(* Logix 5000 AddOnInstructionDefinition export Banner_IOLM_Param_A2_v6; software revision 36.05 *)

TYPE Banner_IOL_Port_v6 :   // UDT that has all of the data items necessary to communicate with a specific Port on a IO-Link Master
STRUCT
   Port_Controlled : INT;   // Each bit represents a port on an IO-Link Master. Set to 1 to tell AOI to control that port.
   Port_Activate : INT;   // Each bit represents a port on an IO-Link Master. When ON that port will process any commands in queue.
   Port_Read : INT;   // Each bit represents a port on an IO-Link Master. Used to determine when device AOI has requested a Read command.
   Port_Write : INT;   // Each bit represents a port on an IO-Link Master. Used to determine when device AOI has requested a Write command.
   Port_RW_Complete : INT;   // Each bit represents a port on an IO-Link Master. Tells device AOI that Read or Write request has been completed.
   Port_Device_Read : INT;
   Data_Transfer : SINT[250];   // Array to transfer data from IO-Master to device AOIs.
END_STRUCT
END_TYPE

TYPE Banner_IOLM_EL_v6 :   // Error Log for Messages to IOLM.
STRUCT
   RW : SINT;   // 0 = Read, 1 = Write.
   Port : SINT;   // Port number that generated error.
   Index : INT;   // IO-Link Index for generated error.
END_STRUCT
END_TYPE

TYPE Banner_IOLM_v6 :   // UDT to control IO-Link Masters.
STRUCT
   Message_Source_Data : SINT[260];
   Message_Destination_Data : SINT[260];
   Error_Log : Banner_IOLM_EL_v6[10];
   Error_Write_Retry : BOOL;
   Num_Error_MSGS : DINT;
   IO_Link_Master_Busy : BOOL;   // 0 = While waiting for a command, 1 = Processing command
   AOI_Reset : BOOL;
   Port_Data : Banner_IOL_Port_v6;   // All of the necessary data to work with the various ports of the IO-Link Master.
   Halt_Operation : BOOL;   // When parameter is 1 the AOI is halted as next available time frame.
   AOI_Halted : BOOL;   // AOI is in standby mode until Halt Operation tag is set back to 0.
END_STRUCT
END_TYPE

ADD_ON_INSTRUCTION Banner_IOLM_Param_A2_v6   (* revision 6.0, vendor Banner Engineering *)
// AOI that controls an Allen Bradley IO-Link Master with Banner devices for parameter data operations. Created for use with the 5032-8IOLM units only.
VAR_IN_OUT
   Message_Read : MESSAGE; {required}   // Message used to gather data from a device plugged into an Allen Bradley IO-Link Master.
   Message_Write : MESSAGE; {required}   // Message used to send parameter updates to a device plugged into an Allen Bradley IO-Link Master.
   IOLM : Banner_IOLM_v6; {required}
   ISDU_Path : STRING[8]; {required}
END_VAR
VAR_INPUT
   Port0 : BOOL; {required}
   Port1 : BOOL; {required}
   Port2 : BOOL; {required}
   Port3 : BOOL; {required}
   Port4 : BOOL; {required}
   Port5 : BOOL; {required}
   Port6 : BOOL; {required}
   Port7 : BOOL; {required}
END_VAR
VAR_OUTPUT
   Done : BOOL; {access Read Only, visible}
   Busy : BOOL; {access Read Only, visible}
   Error : BOOL; {access Read Only, visible}
END_VAR
VAR
   Lock : DINT; {access None}
   Byte_Length : SINT; {access None}
   Current_Port : INT; {access None}   // Current port to communicate with via the IO-Link Master.
   Array_Index : DINT; {access None}
   Data_Index : DINT; {access None}
   Message_Timer : TIMER := (PRE := 100); {access None}
   Error_Index : DINT; {access None}
   Message_Timer2 : TIMER := (PRE := 5000); {access None}
   Temp_Index : INT; {access None}
   Timer8 : TIMER := (PRE := 3000); {access None}
END_VAR

ROUTINE Logic   (* ladder *)
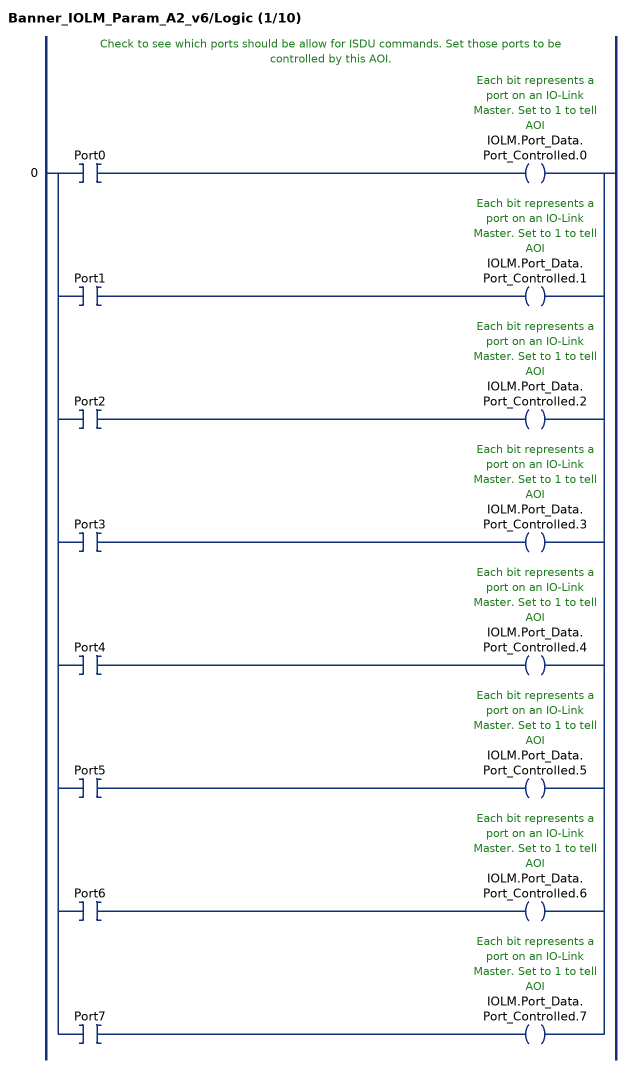
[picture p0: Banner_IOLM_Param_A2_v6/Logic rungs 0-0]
   // Check to see which ports should be allow for ISDU commands. Set those ports to be controlled by this AOI.
   0: [XIC(Port0) OTE(IOLM.Port_Data.Port_Controlled.0) ,XIC(Port1) OTE(IOLM.Port_Data.Port_Controlled.1) ,XIC(Port2) OTE(IOLM.Port_Data.Port_Controlled.2) ,XIC(Port3) OTE(IOLM.Port_Data.Port_Controlled.3) ,XIC(Port4) OTE(IOLM.Port_Data.Port_Controlled.4) ,XIC(Port5) OTE(IOLM.Port_Data.Port_Controlled.5) ,XIC(Port6) OTE(IOLM.Port_Data.Port_Controlled.6) ,XIC(Port7) OTE(IOLM.Port_Data.Port_Controlled.7) ];
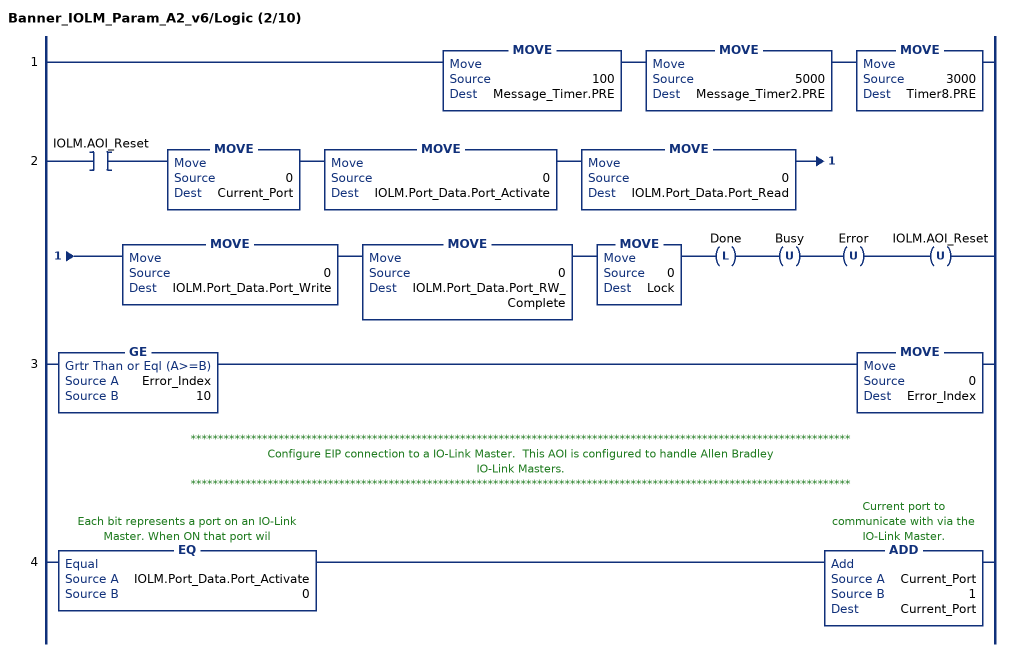
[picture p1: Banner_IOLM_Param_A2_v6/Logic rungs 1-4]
   1: MOVE(100,Message_Timer.PRE)MOVE(5000,Message_Timer2.PRE)MOVE(3000,Timer8.PRE);
   2: XIC(IOLM.AOI_Reset)MOVE(0,Current_Port)MOVE(0,IOLM.Port_Data.Port_Activate)MOVE(0,IOLM.Port_Data.Port_Read)MOVE(0,IOLM.Port_Data.Port_Write)MOVE(0,IOLM.Port_Data.Port_RW_Complete)MOVE(0,Lock)OTL(Done)OTU(Busy)OTU(Error)OTU(IOLM.AOI_Reset);
   3: GE(Error_Index,10)MOVE(0,Error_Index);
   // ************************************************************************************************************************
   // Configure EIP connection to a IO-Link Master.  This AOI is configured to handle Allen Bradley
   // IO-Link Masters.
   // ************************************************************************************************************************
   4: EQ(IOLM.Port_Data.Port_Activate,0)ADD(Current_Port,1,Current_Port);
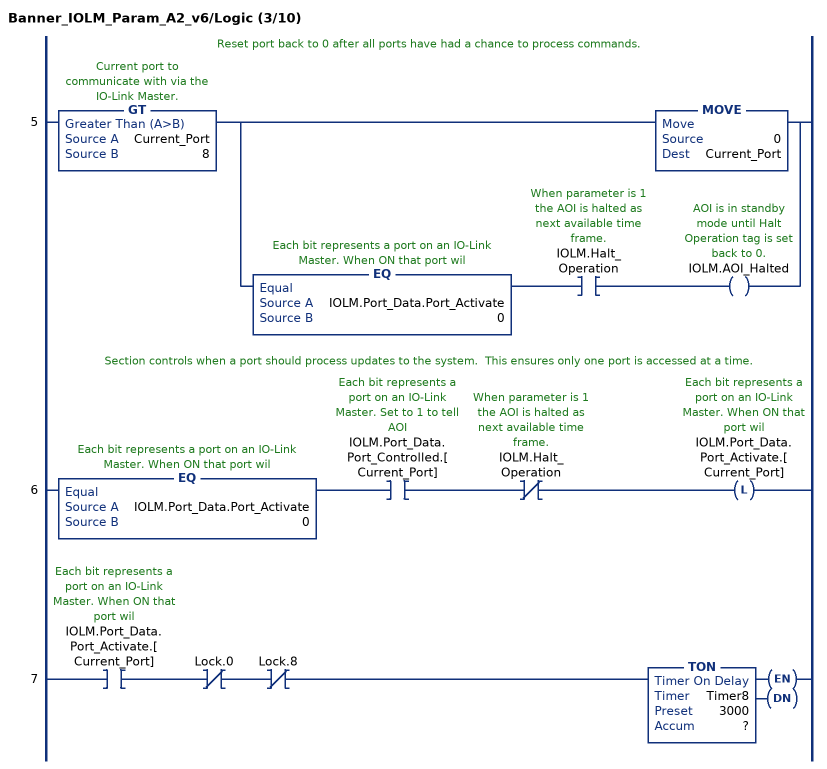
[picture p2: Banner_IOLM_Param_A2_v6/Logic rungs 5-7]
   // Reset port back to 0 after all ports have had a chance to process commands.
   5: GT(Current_Port,8)[MOVE(0,Current_Port) ,EQ(IOLM.Port_Data.Port_Activate,0) XIC(IOLM.Halt_Operation) OTE(IOLM.AOI_Halted) ];
   // Section controls when a port should process updates to the system.  This ensures only one port is accessed at a time.
   6: EQ(IOLM.Port_Data.Port_Activate,0)XIC(IOLM.Port_Data.Port_Controlled.[Current_Port])XIO(IOLM.Halt_Operation)OTL(IOLM.Port_Data.Port_Activate.[Current_Port]);
   7: XIC(IOLM.Port_Data.Port_Activate.[Current_Port])XIO(Lock.0)XIO(Lock.8)TON(Timer8,?,?);
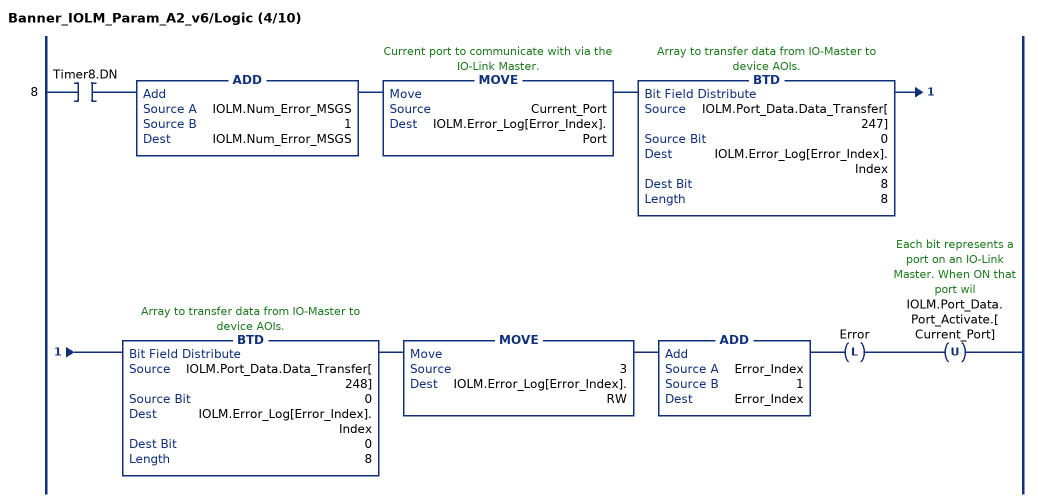
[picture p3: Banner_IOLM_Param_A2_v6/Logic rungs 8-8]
   8: XIC(Timer8.DN)ADD(IOLM.Num_Error_MSGS,1,IOLM.Num_Error_MSGS)MOVE(Current_Port,IOLM.Error_Log[Error_Index].Port)BTD(IOLM.Port_Data.Data_Transfer[247],0,IOLM.Error_Log[Error_Index].Index,8,8)BTD(IOLM.Port_Data.Data_Transfer[248],0,IOLM.Error_Log[Error_Index].Index,0,8)MOVE(3,IOLM.Error_Log[Error_Index].RW)ADD(Error_Index,1,Error_Index)OTL(Error)OTU(IOLM.Port_Data.Port_Activate.[Current_Port]);
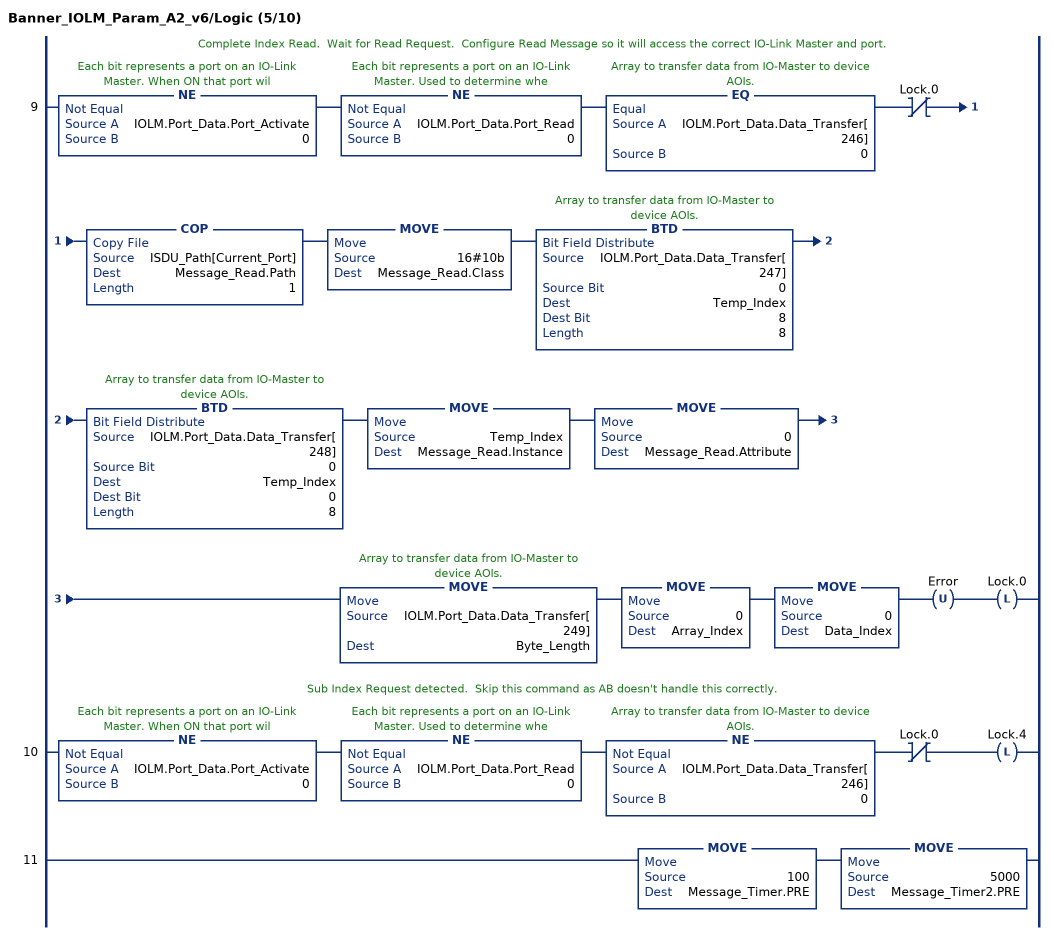
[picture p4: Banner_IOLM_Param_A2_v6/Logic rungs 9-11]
   // Complete Index Read.  Wait for Read Request.  Configure Read Message so it will access the correct IO-Link Master and port.
   9: NE(IOLM.Port_Data.Port_Activate,0)NE(IOLM.Port_Data.Port_Read,0)EQ(IOLM.Port_Data.Data_Transfer[246],0)XIO(Lock.0)COP(ISDU_Path[Current_Port],Message_Read.Path,1)MOVE(16#10b,Message_Read.Class)BTD(IOLM.Port_Data.Data_Transfer[247],0,Temp_Index,8,8)BTD(IOLM.Port_Data.Data_Transfer[248],0,Temp_Index,0,8)MOVE(Temp_Index,Message_Read.Instance)MOVE(0,Message_Read.Attribute)MOVE(IOLM.Port_Data.Data_Transfer[249],Byte_Length)MOVE(0,Array_Index)MOVE(0,Data_Index)OTU(Error)OTL(Lock.0);
   // Sub Index Request detected.  Skip this command as AB doesn't handle this correctly.
   10: NE(IOLM.Port_Data.Port_Activate,0)NE(IOLM.Port_Data.Port_Read,0)NE(IOLM.Port_Data.Data_Transfer[246],0)XIO(Lock.0)OTL(Lock.4);
   11: MOVE(100,Message_Timer.PRE)MOVE(5000,Message_Timer2.PRE);
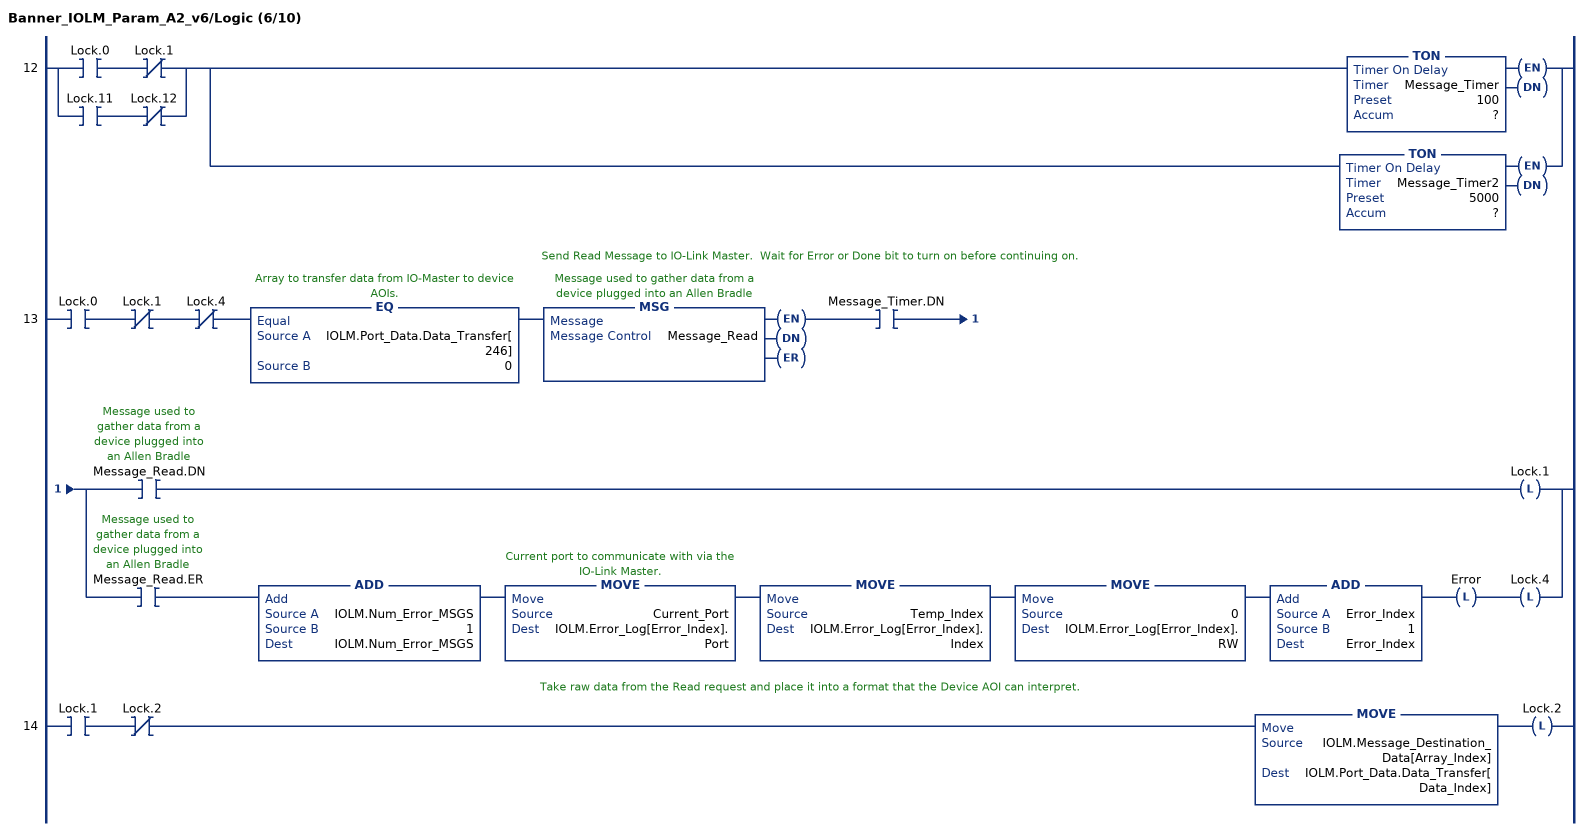
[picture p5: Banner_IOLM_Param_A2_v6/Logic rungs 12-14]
   12: [XIC(Lock.0) XIO(Lock.1) ,XIC(Lock.11) XIO(Lock.12) ][TON(Message_Timer,?,?) ,TON(Message_Timer2,?,?) ];
   // Send Read Message to IO-Link Master.  Wait for Error or Done bit to turn on before continuing on.
   13: XIC(Lock.0)XIO(Lock.1)XIO(Lock.4)EQ(IOLM.Port_Data.Data_Transfer[246],0)MSG(Message_Read)XIC(Message_Timer.DN)[XIC(Message_Read.DN) OTL(Lock.1) ,XIC(Message_Read.ER) ADD(IOLM.Num_Error_MSGS,1,IOLM.Num_Error_MSGS) MOVE(Current_Port,IOLM.Error_Log[Error_Index].Port) MOVE(Temp_Index,IOLM.Error_Log[Error_Index].Index) MOVE(0,IOLM.Error_Log[Error_Index].RW) ADD(Error_Index,1,Error_Index) OTL(Error) OTL(Lock.4) ];
   // Take raw data from the Read request and place it into a format that the Device AOI can interpret.
   14: XIC(Lock.1)XIO(Lock.2)MOVE(IOLM.Message_Destination_Data[Array_Index],IOLM.Port_Data.Data_Transfer[Data_Index])OTL(Lock.2);
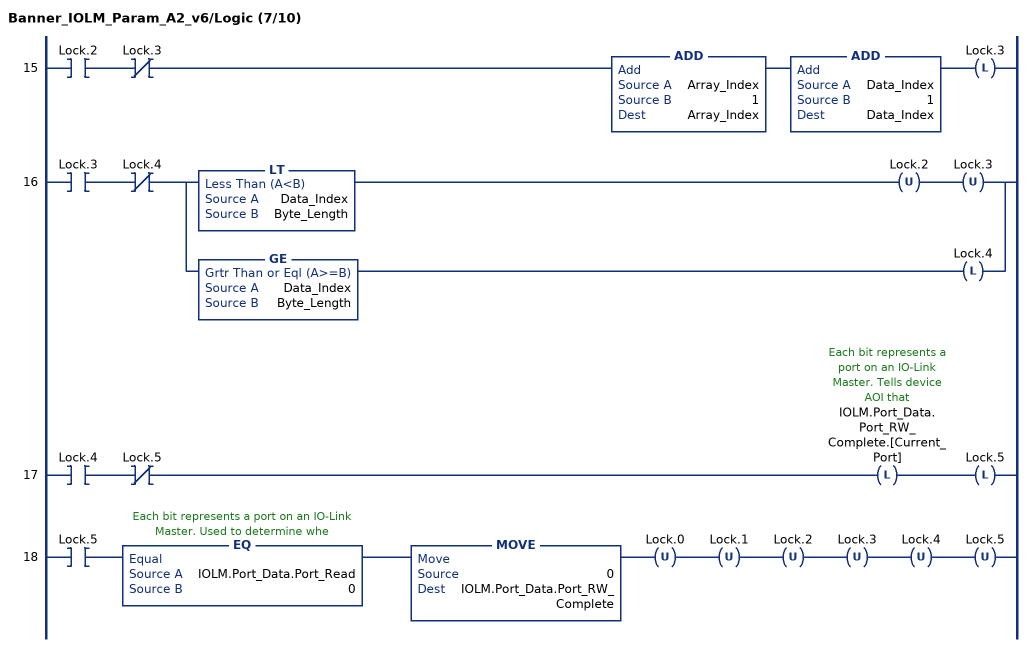
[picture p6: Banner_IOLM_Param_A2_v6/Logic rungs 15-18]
   15: XIC(Lock.2)XIO(Lock.3)ADD(Array_Index,1,Array_Index)ADD(Data_Index,1,Data_Index)OTL(Lock.3);
   16: XIC(Lock.3)XIO(Lock.4)[LT(Data_Index,Byte_Length) OTU(Lock.2) OTU(Lock.3) ,GE(Data_Index,Byte_Length) OTL(Lock.4) ];
   17: XIC(Lock.4)XIO(Lock.5)OTL(IOLM.Port_Data.Port_RW_Complete.[Current_Port])OTL(Lock.5);
   18: XIC(Lock.5)EQ(IOLM.Port_Data.Port_Read,0)MOVE(0,IOLM.Port_Data.Port_RW_Complete)OTU(Lock.0)OTU(Lock.1)OTU(Lock.2)OTU(Lock.3)OTU(Lock.4)OTU(Lock.5);
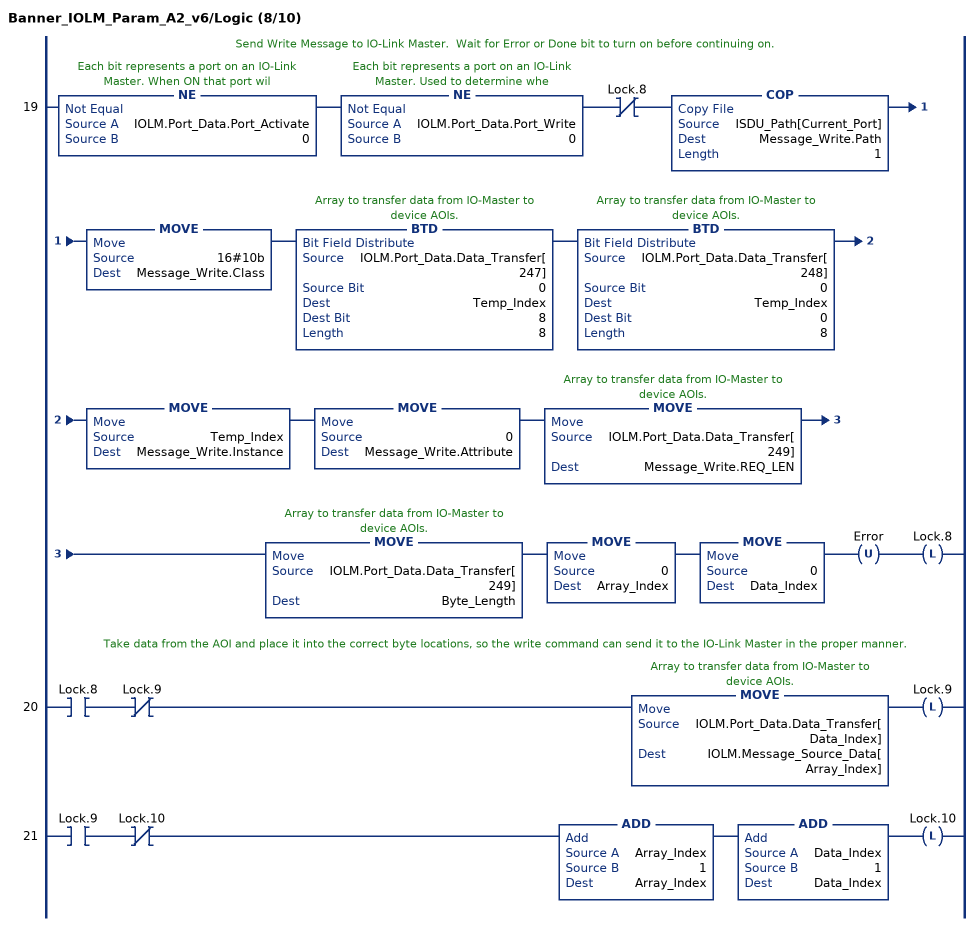
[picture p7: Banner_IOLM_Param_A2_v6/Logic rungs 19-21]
   // Send Write Message to IO-Link Master.  Wait for Error or Done bit to turn on before continuing on.
   19: NE(IOLM.Port_Data.Port_Activate,0)NE(IOLM.Port_Data.Port_Write,0)XIO(Lock.8)COP(ISDU_Path[Current_Port],Message_Write.Path,1)MOVE(16#10b,Message_Write.Class)BTD(IOLM.Port_Data.Data_Transfer[247],0,Temp_Index,8,8)BTD(IOLM.Port_Data.Data_Transfer[248],0,Temp_Index,0,8)MOVE(Temp_Index,Message_Write.Instance)MOVE(0,Message_Write.Attribute)MOVE(IOLM.Port_Data.Data_Transfer[249],Message_Write.REQ_LEN)MOVE(IOLM.Port_Data.Data_Transfer[249],Byte_Length)MOVE(0,Array_Index)MOVE(0,Data_Index)OTU(Error)OTL(Lock.8);
   // Take data from the AOI and place it into the correct byte locations, so the write command can send it to the IO-Link Master in the proper manner.
   20: XIC(Lock.8)XIO(Lock.9)MOVE(IOLM.Port_Data.Data_Transfer[Data_Index],IOLM.Message_Source_Data[Array_Index])OTL(Lock.9);
   21: XIC(Lock.9)XIO(Lock.10)ADD(Array_Index,1,Array_Index)ADD(Data_Index,1,Data_Index)OTL(Lock.10);
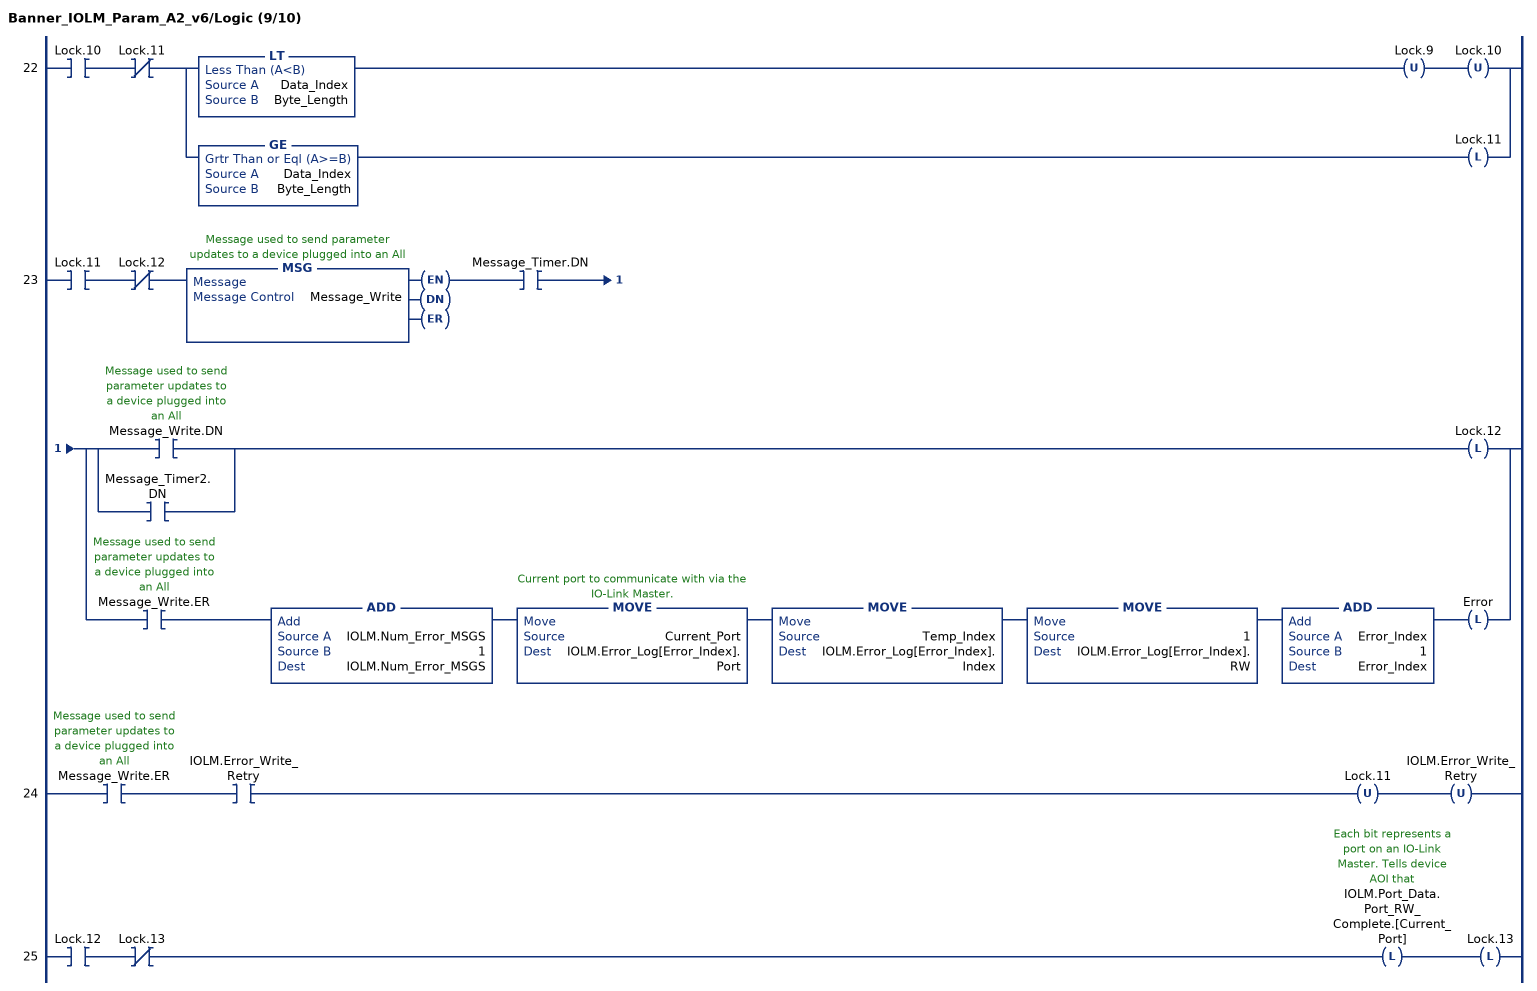
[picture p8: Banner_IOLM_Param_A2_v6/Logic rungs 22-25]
   22: XIC(Lock.10)XIO(Lock.11)[LT(Data_Index,Byte_Length) OTU(Lock.9) OTU(Lock.10) ,GE(Data_Index,Byte_Length) OTL(Lock.11) ];
   23: XIC(Lock.11)XIO(Lock.12)MSG(Message_Write)XIC(Message_Timer.DN)[[XIC(Message_Write.DN) ,XIC(Message_Timer2.DN) ] OTL(Lock.12) ,XIC(Message_Write.ER) ADD(IOLM.Num_Error_MSGS,1,IOLM.Num_Error_MSGS) MOVE(Current_Port,IOLM.Error_Log[Error_Index].Port) MOVE(Temp_Index,IOLM.Error_Log[Error_Index].Index) MOVE(1,IOLM.Error_Log[Error_Index].RW) ADD(Error_Index,1,Error_Index) OTL(Error) ];
   24: XIC(Message_Write.ER)XIC(IOLM.Error_Write_Retry)OTU(Lock.11)OTU(IOLM.Error_Write_Retry);
   25: XIC(Lock.12)XIO(Lock.13)OTL(IOLM.Port_Data.Port_RW_Complete.[Current_Port])OTL(Lock.13);
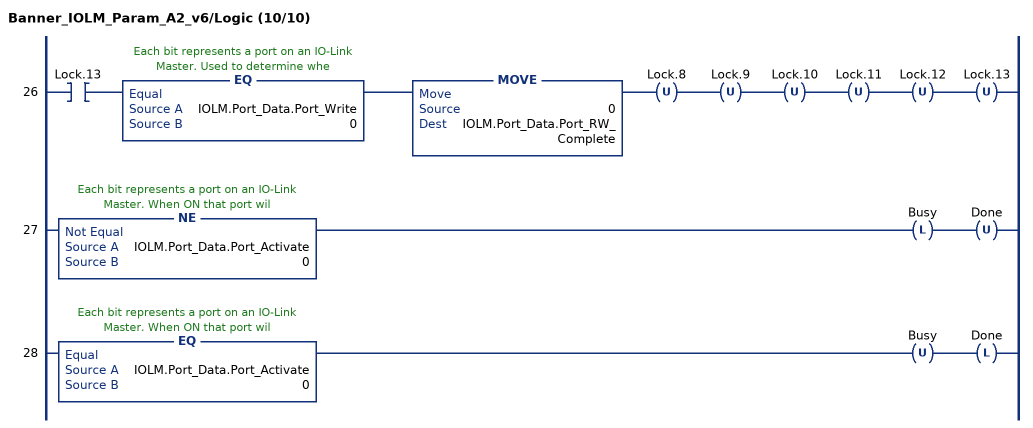
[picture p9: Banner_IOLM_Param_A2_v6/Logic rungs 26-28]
   26: XIC(Lock.13)EQ(IOLM.Port_Data.Port_Write,0)MOVE(0,IOLM.Port_Data.Port_RW_Complete)OTU(Lock.8)OTU(Lock.9)OTU(Lock.10)OTU(Lock.11)OTU(Lock.12)OTU(Lock.13);
   27: NE(IOLM.Port_Data.Port_Activate,0)OTL(Busy)OTU(Done);
   28: EQ(IOLM.Port_Data.Port_Activate,0)OTU(Busy)OTL(Done);
END_ROUTINE
END_ADD_ON_INSTRUCTION
